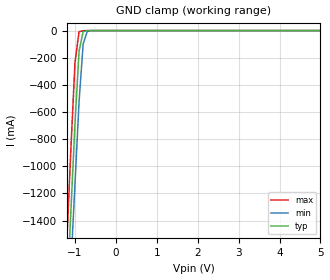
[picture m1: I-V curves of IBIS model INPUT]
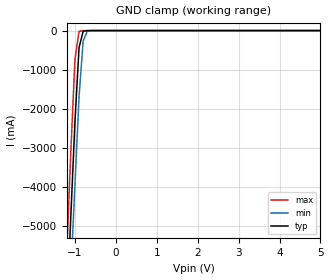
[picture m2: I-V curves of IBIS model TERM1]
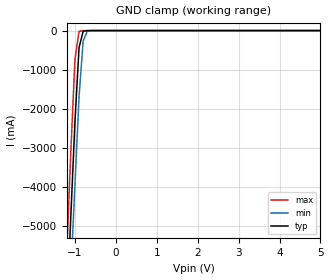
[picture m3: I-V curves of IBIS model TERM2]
|   PERICOM SEMICONDUCTOR CORP
|   IBIS Model of PI5C3126
|   Product Family: 5C
|   QSOP (Q) Package
[IBIS Ver] 3.2
[Comment char] |_char
[File Name] pi5c3126_q_50v.ibs
[File Rev] 1.0
[Source] File originated at Pericom Semiconductor Corp.
[Date] 05/09/14
[Disclaimer] (C) Copyright PERICOM Semiconductor Corporation
   All rights reserved
  Pericom Semiconductor Corporation hereby grants the user of
  this IBIS model a non-exclusive, nontransferable license to
  use this IBIS model under the following terms.
  This IBIS model is provided on an "AS IS" basis and Pericom
  makes absolutely no warranty with respect to the information
  contained herein. PERICOM DISCLAIMS AND CUSTOMER WAIVES ALL
  WARRANTIES, EXPRESSED OR IMPLIED, INCLUDING WARRANTIES OF
  MERCHANTABILITY OR FITNESS FOR A PARTICULAR PURPOSE. The
  entire risk as to quality and performance is with the customer.
  Accordingly, in no event shall the company be liable for any
  damages, whether in contract or tort, including any lost
  profits or other incidental, consequential, exemplary, or
  punitive damages arising out of the use or application of the
  IBIS model provided in this package. Further, Pericom reserves
  the right to make changes without notice to any product herein
  to improve reliability, function, or design. Pericom does not
  convey any license under patent rights or any other intellectual
  property rights, including those of third parties.
  The user is granted this license only to use the IBIS model
  and is not granted rights to sell, load, rent, lease or license
  the IBIS model in whole or in part, or in modified form to anyone
  other than user. User may modify the IBIS model to suit its specific
  application but rights to derivative works and such modifications
  shall belong to Pericom.
  Pericom is not obligated to provide maintenance or support
  for the licensed IBIS model.
  Contact Pericom at ATTN: APPLICATION ENGINEERING / IBIS MODELS
  1545 Barber Lane Milpitas, CA 95035 USA.
[Component] PI5C3126
[Manufacturer] Pericom Semiconductor Corp.
[Package]
| variable   typ   min  max
R_pkg   0.04446ohm   NA   NA
L_pkg   2.45300nH   NA   NA
C_pkg   0.36900pF   NA   NA
[Pin] signal_name   model_name   R_pin   L_pin   C_pin
1   NC   NC   0.04491   2.77500nH   0.44400pF
2   BE0   INPUT   0.04461   2.56033nH   0.39400pF
3   A0   TERM1   0.04431   2.34567nH   0.34400pF
4   B0   TERM2   0.04401   2.13100nH   0.29400pF
5   BE1   INPUT   0.04401   2.13100nH   0.29400pF
6   A1   TERM1   0.04431   2.34567nH   0.34400pF
7   B1   TERM2   0.04461   2.56033nH   0.39400pF
8   GND   GND   0.04491   2.77500nH   0.44400pF
9   NC   NC   0.04491   2.77500nH   0.44400pF
10   B2   TERM1   0.04461   2.56033nH   0.39400pF
11   A2   TERM1   0.04431   2.34567nH   0.34400pF
12   BE2   INPUT   0.04401   2.13100nH   0.29400pF
13   B3   TERM2   0.04401   2.13100nH   0.29400pF
14   A3   TERM1   0.04431   2.34567nH   0.34400pF
15   BE3   INPUT   0.04461   2.56033nH   0.39400pF
16   VCC   POWER   0.04491   2.77500nH   0.44400pF
[Series Switch Groups]
On 1 /
[Series_Pin_Mapping]   pin_2   model_name   function_table_group
4   3   SWITCH1   1
7   6   SWITCH1   1
10   11   SWITCH1   1
13   14   SWITCH1   1
|   Model SWITCH1
[Model] SWITCH1
Model_type Series_switch
| variable   typ   min   max
C_comp   8.0000pF   7.9200pF   8.0800pF
[Voltage Range]   5.0000V   4.5000V   5.5000V
[temperature range]   25   85   -40
[On]
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[OFF]
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| Models and submodels in the file (4): INPUT (Input), SWITCH1 (Series_switch), TERM1 (Terminator), TERM2 (Terminator)
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|   Model INPUT
[Model] INPUT
Model_type Input
Vinl = 1.500V
Vinh = 3.500V
| variable   typ   min   max
C_comp   6.0000pF   5.9400pF   6.0600pF
[Voltage Range]   5.0000V   4.5000V   5.5000V
[temperature range]   25   85   -40
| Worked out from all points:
|   GND clamp passes 1 mA (typ) near -0.71 V on its own axis
[GND Clamp]
| Voltage   I(typ)   I(min)   I(max)
-5V       -26.43A    -25.51A    -27.59A
-1.2V     -1.976A    -2.351A    -1.561A
-1.1V     -1.333A    -1.742A    -876.1mA
-1V       -689.5mA   -1.133A    -237.7mA
-900mV    -152.8mA   -525.5mA   -8.619mA
-800mV    -7.512mA   -99.97mA   -842.8uA
-700mV    -518.9uA   -6.478mA   -104.3uA
-500mV    -3.741uA   -32.95uA   -179.2nA
5V        81.04pA    180.4pA    80.01pA
[POWER Clamp]
| Voltage   I(typ)   I(min)   I(max)
-5V       0A         0A         0A
0V        0A         0A         0A
|   Model TERM1
[Model] TERM1
Model_type Terminator
| variable   typ   min   max
C_comp   6.0000pF   5.9400pF   6.0600pF
[Voltage Range]   5.0000V   4.5000V   5.5000V
[temperature range]   25   85   -40
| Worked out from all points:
|   GND clamp passes 1 mA (typ) near -0.69 V on its own axis
[GND Clamp]
| Voltage   I(typ)   I(min)   I(max)
-5V       -98.4A     -94.6A     -103.2A
-1.2V     -7.136A    -8.475A    -5.649A
-1.1V     -4.734A    -6.209A    -3.081A
-1V       -2.333A    -3.943A    -732.6mA
-900mV    -436.8mA   -1.694A    -20.9mA
-800mV    -19.19mA   -272.2mA   -1.375mA
-700mV    -1.088mA   -17.12mA   -157.3uA
-500mV    -5.777uA   -75.55uA   -268.9nA
5V        184pA      267.6pA    183.2pA
[POWER Clamp]
| Voltage   I(typ)   I(min)   I(max)
-5V       0A         0A         0A
0V        0A         0A         0A
|   Model TERM2
[Model] TERM2
Model_type Terminator
| variable   typ   min   max
C_comp   6.0000pF   5.9400pF   6.0600pF
[Voltage Range]   5.0000V   4.5000V   5.5000V
[temperature range]   25   85   -40
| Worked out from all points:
|   GND clamp passes 1 mA (typ) near -0.69 V on its own axis
[GND Clamp]
| Voltage   I(typ)   I(min)  I(max)
-5V       -98.4A     -94.6A     -103.2A
-1.2V     -7.136A    -8.475A    -5.649A
-1.1V     -4.734A    -6.209A    -3.081A
-1V       -2.333A    -3.943A    -732.6mA
-900mV    -436.8mA   -1.694A    -20.9mA
-800mV    -19.19mA   -272.2mA   -1.375mA
-700mV    -1.088mA   -17.12mA   -157.3uA
-500mV    -5.777uA   -75.55uA   -268.9nA
5V        184pA      267.5pA    183.2pA
[POWER Clamp]
| Voltage   I(typ)   I(min)   I(max)
-5V       0A         0A         0A
0V        0A         0A         0A
